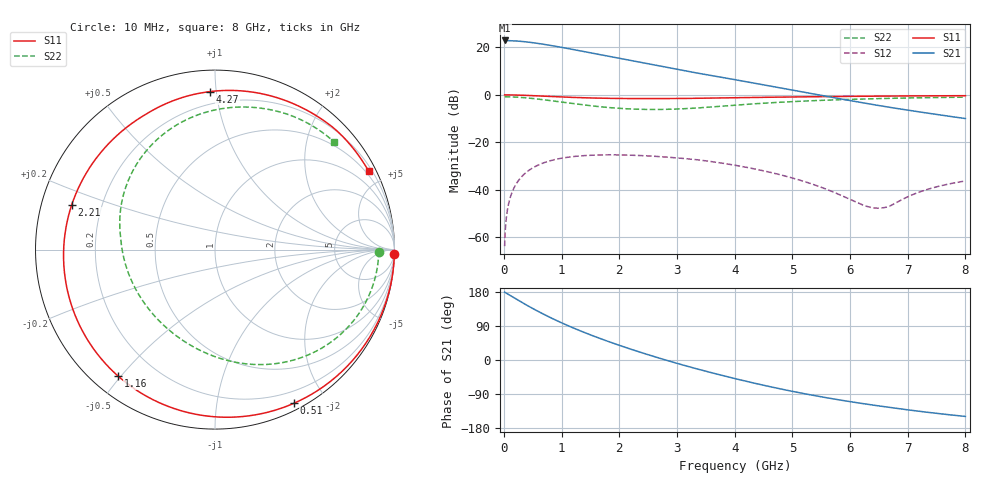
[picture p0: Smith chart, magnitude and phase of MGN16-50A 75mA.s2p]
! Port[1] = GATE
! Port[2] = DRAIN
! [Type]  S-parameter s2p file touchstone ver. 1.0
! [Object]  MGN16-50A
! [Bias]  75 mA
! [Version]  1.0
! [Date]  Thu May 28 10:54:03 2026
! [Source]  This file was created in JSC "ICC Milandr".
! [Disclaimer] Property of JSC "ICC Milandr". Unauthorized reproduction and/or distribution is strictly prohibited.
!  The file and the data are provided "AS IS" and with all faults and disclaim all warranties, express and implied, including
!  without limitation any implied warranties of merchantability, fitness for a particular purpose.
!  JSC "ICC Milandr" assumes no liability for:
!  1) the accuracy of the data provided;
!  2) the proper functioning of this data;
!  3) infringement of patents, copyrights or intellectual property rights resulting from the use of this data.
!  JSC "ICC Milandr" reserves the right to make changes to the products and the data without prior notice.
!  Please, be aware that your receipt and use of the file provided shall serve as acceptance of these terms and conditions.
!  If you do not accept these terms, you should return or destroy this file and any other accompanying information immediately.
# hz S ma R 12.5
! 2 Port Network Data from SP1.SP block
! freq  magS11  angS11  magS21  angS21  magS12  angS12  magS22  angS22
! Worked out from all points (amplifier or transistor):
!   800 points, 10 MHz to 8 GHz, reference 12.5 ohm
!   highest |S21| = 22.9 dB at 10 MHz (marker M1)
!   |S21| within 3 dB of that: start of sweep to 1.019 GHz
!   unconditionally stable (mu >= 1): 4.372 GHz to end of sweep
!   at 1.34 GHz: K = 0.18, MSG = 22.0 dB, |S12| = -25.6 dB
!   at 4.01 GHz: K = 0.82, MSG = 18.0 dB, |S12| = -29.6 dB
!   at 8 GHz: K = 1.41, MAG = 9.3 dB, |S12| = -36.2 dB
!   S11 on the Smith chart (normalised r, x): 10 MHz: 2, -90; 510 MHz: 0.07, -1.63; 1.16 GHz: 0.07, -0.49; 2.21 GHz: 0.09, +0.15; 4.27 GHz: 0.12, +0.96; 8 GHz: 0.36, +4.13
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1e7  0.9995 -1.3  13.96 179.0  0.000656 82.5  0.9122 -0.7
9e7  0.9981 -11.6  13.88 171.7  0.005819 81.3  0.9095 -6.6
2.3e8  0.9906 -29.3  13.58 159.0  0.01455 69.6  0.8948 -16.8
3.7e8  0.9781 -46.5  13.09 146.7  0.02259 57.9  0.8695 -26.6
5.1e8  0.9624 -62.9  12.48 134.9  0.02969 46.7  0.8368 -36.0
6.5e8  0.9453 -78.4  11.79 123.6  0.03576 36.1  0.7998 -44.9
8e8  0.9268 -94.0  11.02 112.2  0.04112 25.3  0.7582 -53.9
9.7e8  0.9071 -110.5  10.14 100.0  0.04587 13.8  0.7118 -63.6
1.16e9  0.8878 -127.4  9.193 87.3  0.04974 1.7  0.6634 -73.9
1.35e9  0.8719 -142.8  8.317 75.2  0.05234 -9.6  0.6203 -83.9
1.54e9  0.8592 -156.9  7.516 63.9  0.05391 -20.2  0.5835 -93.6
1.74e9  0.8491 -170.3  6.755 52.6  0.05466 -30.8  0.5517 -103.7
1.96e9  0.8414 176.2  6.008 40.8  0.05465 -41.9  0.5249 -115.0
2.21e9  0.8362 162.6  5.262 28.0  0.0538 -53.9  0.5045 -127.9
2.68e9  0.835 140.8  4.106 5.5  0.05042 -75.2  0.4936 -152.7
2.97e9  0.8387 129.4  3.522 -7.5  0.04753 -87.5  0.5028 -168.0
3.27e9  0.8452 119.0  3.002 -20.3  0.04409 -99.8  0.5226 176.7
4.01e9  0.8721 98.2  2.083 -49.3  0.033 -122.5  0.6091 144.3
4.27e9  0.8811 91.7  1.828 -58.7  0.02886 -129.3  0.6409 134.1
5.34e9  0.9135 68.3  1.057 -92.7  0.01332 -148.3  0.7535 98.3
6.67e9  0.9468 45.6  0.5508 -124.7  0.00445 -83.3  0.8449 65.8
8e9  0.9613 27.1  0.3178 -148.9  0.01546 -60.5  0.8948 42.2
